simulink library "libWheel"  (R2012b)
settings: Solver=ode45  StartTime=0.0  StopTime=10.0  RelTol=1e-3
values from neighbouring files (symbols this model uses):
  WR = 0.25    [initWheel.m]    (also in initVehicle.m)

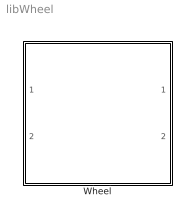
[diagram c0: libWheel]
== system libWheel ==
  Wheel : Subsystem

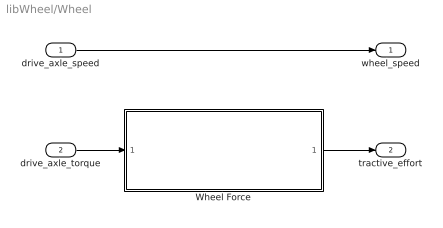
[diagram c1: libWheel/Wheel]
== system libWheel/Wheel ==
  drive_axle_speed : Inport
  drive_axle_torque : Inport  Port=2
  Wheel Force : Subsystem
  wheel_speed : Outport
  tractive_effort : Outport  Port=2
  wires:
  Wheel Force/1(tractive_effort) -> tractive_effort/1
  drive_axle_torque/1 -> Wheel Force/1(drive_axle_torque)
  drive_axle_speed/1 -> wheel_speed/1

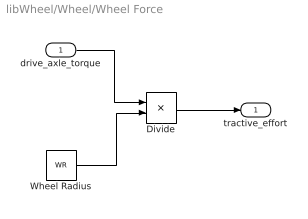
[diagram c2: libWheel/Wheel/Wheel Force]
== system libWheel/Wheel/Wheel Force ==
  drive_axle_torque : Inport
  Divide : Product  Inputs=*/
  Wheel Radius : Constant  Value=WR
  tractive_effort : Outport
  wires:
  drive_axle_torque/1 -> Divide/1
  Wheel Radius/1 -> Divide/2
  Divide/1 -> tractive_effort/1
